| IBIS file stm32u535_545_wlcsp56_smps.ibs
[IBIS ver] 4.2
[File name] stm32u535_545_wlcsp56_smps.ibs
[File Rev] rev1.0
[Date]  11-09-2023
[Source] Data Created at STMicroelectronics
[Notes]  File originated from ELDO simulations.
[Disclaimer]  This information is for modeling purpose only and is
   not guaranteed. The information is subject to change without
   notice.
[Copyright] Copyright 2023 STMicroelectronics Inc.
|   Component stm32u535_545_wlcsp56_smps
[Component] stm32u535_545_wlcsp56_smps
[Manufacturer] STMicroelectronics
[Package]
| variable   typ   min   max
R_pkg  0  NA  NA
L_pkg  0  NA  NA
C_pkg  0  NA  NA
[Pin]   signal_name   model_name
A1  VDDUSB  power
A3  PA15  io8_100m_ft
A5  PA14  io8_100m_ft
A7  PB5  io8_166m_hslv_ft
A9  PB8  io8_100m_hslv_i2c_ft
A11  VDD11  nc
A13  VDD  power
B2  VSS  gnd
B4  PB3  io8_100m_i2c_ft
B6  PB4  io8_100m_i2c_ft
B8  PH3-BOOT0  io8_100m_ft
B10  VSS  gnd
B12  PE4  io8_100m_hslv_tamp_ft
B14  VBAT  power
C1  PA11  io8_usb_ft
C3  PA12  io8_usb_ft
C5  PA13  io8_100m_ft
C7  PB6  io8_100m_i2c_ft
C9  PB9  io8_100m_hslv_i2c_ft
C11  PE3  io8_100m_hslv_tamp_ft
C13  PC14-OSC32_IN  io8_100m_tamp_ft
D2  PA9  io8_100m_ft
D4  PA10  io8_100m_ft
D6  PA3  io8_166m_hslv_ft
D8  PB7  io8_166m_hslv_i2c_ft
D10  PE5  io8_100m_hslv_tamp_ft
D12  PC13  io8_100m_ft_v33
D14  PC15-OSC32_OUT   io8_100m_tamp_ft
E1  PB14  io8_100m_i2c_ft
E3  PB12  io8_166m_hslv_ft
E5  PA8  io8_166m_hslv_ft
E7  PA2  io8_100m_hslv_ft
E9  NRST  nc
E11  PH1-OSC_OUT  io8_100m_ft
E13  PH0-OSC_IN  io8_100m_ft
F2  PB15  io8_100m_ft
F4  PB1  io8_100m_hslv_ft
F6  PB0  io8_100m_hslv_ft
F8  PA5  io8_100m_ft
F10  PA0  io8_100m_hslv_tamp_ft
F12  VDDA  power
F14  VSSA  nc
G1  PB13  io8_100m_i2c_ft
G3  VSS  gnd
G5  VSSSMPS  nc
G7  PB2  io8_100m_hslv_tamp_ft
G9  PA6  io8_100m_hslv_ft
G11  PA4  io8_100m_hslv_ft
G13  PA1  io8_100m_hslv_tamp_ft
H2  VDD  power
H4  VDD11  nc
H6  VDDSMPS  nc
H8  VLXSMPS  nc
H10  PA7  io8_100m_hslv_i2c_ft
H12  VDD  power
H14  VSS  gnd
[Package Model]   455-wlcsp-56-100mhz-230421
[Pin Mapping]   pulldown_ref   pullup_ref   | Comment
A1  nc  vddiom
A3  gndio  vddiom
A5  gndio  vddiom
A7  gndio  vddiom
A9  gndio  vddiom
A11  nc  nc
A13  nc  vddiom
B2  gndio  nc
B4  gndio  vddiom
B6  gndio  vddiom
B8  gndio  vddiom
B10  gndio  nc
B12  gndio  vddiom
B14  nc  vsw
C1  gndio  vddiom
C3  gndio  vddiom
C5  gndio  vddiom
C7  gndio  vddiom
C9  gndio  vddiom
C11  gndio  vddiom
C13  gndio  vddiom  | Depending on IO usage
| C13  gndio  vsw  | Depending on IO usage
D2  gndio  vddiom
D4  gndio  vddiom
D6  gndio  vddiom
D8  gndio  vddiom
D10  gndio  vddiom
D12  gndio  vddiom  | Depending on IO usage
| D12  gndio  vsw  | Depending on IO usage
D14  gndio  vddiom  | Depending on IO usage
| D14  gndio  vsw  | Depending on IO usage
E1  gndio  vddiom
E3  gndio  vddiom
E5  gndio  vddiom
E7  gndio  vddiom
E9  nc   nc
E11  gndio  vddiom
E13  gndio  vddiom
F2  gndio  vddiom
F4  gndio  vddiom
F6  gndio  vddiom
F8  gndio  vddiom
F10  gndio  vddiom
F12  nc  vddiom
F14  nc  nc
G1  gndio  vddiom
G3  gndio  nc
G5  nc  nc
G7  gndio  vddiom
G9  gndio  vddiom
G11  gndio  vddiom
G13  gndio  vddiom
H2  nc  vddiom
H4  nc  nc
H6  nc  nc
H8  nc  nc
H10  gndio  vddiom
H12  nc  vddiom
H14  gndio  nc
[Model Selector] io8_100m_ft
io8_100m_ft_hs_1v2  "IO8_FT 100MHz high speed @ 1.2V"
io8_100m_ft_fs_1v2  "IO8_FT 100MHz fast speed @ 1.2V"
io8_100m_ft_fs_pd_1v2  "IO8_FT 100MHz fast speed @ 1.2V pulldown"
io8_100m_ft_ms_1v2  "IO8_FT 100MHz med speed @ 1.2V"
io8_100m_ft_ms_pd_1v2  "IO8_FT 100MHz med speed @ 1.2V pulldown"
io8_100m_ft_ls_1v2  "IO8_FT 100MHz low speed @ 1.2V"
io8_100m_ft_ls_pd_1v2  "IO8_FT 100MHz low speed @ 1.2V pulldown"
io8_100m_ft_hs_1v8  "IO8_FT 100MHz high speed @ 1.8V"
io8_100m_ft_hs_pd_1v8  "IO8_FT 100MHz high speed @ 1.8V pulldown"
io8_100m_ft_fs_1v8  "IO8_FT 100MHz fast speed @ 1.8V"
io8_100m_ft_fs_pd_1v8  "IO8_FT 100MHz fast speed @ 1.8V pulldown"
io8_100m_ft_ms_1v8  "IO8_FT 100MHz med speed @ 1.8V"
io8_100m_ft_ms_pd_1v8  "IO8_FT 100MHz med speed @ 1.8V pulldown"
io8_100m_ft_ls_1v8  "IO8_FT 100MHz low speed @ 1.8V"
io8_100m_ft_ls_pd_1v8  "IO8_FT 100MHz low speed @ 1.8V pulldown"
io8_100m_ft_hs_3v3  "IO8_FT 100MHz high speed @ 3.3V"
io8_100m_ft_hs_pd_3v3  "IO8_FT 100MHz high speed @ 3.3V pulldown"
io8_100m_ft_fs_3v3  "IO8_FT 100MHz fast speed @ 3.3V"
io8_100m_ft_fs_pd_3v3  "IO8_FT 100MHz fast speed @ 3.3V pulldown"
io8_100m_ft_ms_3v3  "IO8_FT 100MHz med speed @ 3.3V"
io8_100m_ft_ms_pd_3v3  "IO8_FT 100MHz med speed @ 3.3V pulldown"
io8_100m_ft_ls_3v3  "IO8_FT 100MHz low speed @ 3.3V"
io8_100m_ft_ls_pd_3v3  "IO8_FT 100MHz low speed @ 3.3V pulldown"
[Model Selector] io8_100m_hslv_ft
io8_100m_ft_hs_1v2  "IO8_FT 100MHz high speed @ 1.2V"
io8_100m_ft_hs_pu_1v2  "IO8_FT 100MHz high speed @ 1.2V pullup"
io8_100m_ft_hs_pd_1v2  "IO8_FT 100MHz high speed @ 1.2V pulldown"
io8_100m_ft_fs_1v2  "IO8_FT 100MHz fast speed @ 1.2V"
io8_100m_ft_fs_pu_1v2  "IO8_FT 100MHz fast speed @ 1.2V pullup"
io8_100m_ft_fs_pd_1v2  "IO8_FT 100MHz fast speed @ 1.2V pulldown"
io8_100m_ft_ms_1v2  "IO8_FT 100MHz med speed @ 1.2V"
io8_100m_ft_ms_pu_1v2  "IO8_FT 100MHz med speed @ 1.2V pullup"
io8_100m_ft_ms_pd_1v2  "IO8_FT 100MHz med speed @ 1.2V pulldown"
io8_100m_ft_ls_1v2  "IO8_FT 100MHz low speed @ 1.2V"
io8_100m_ft_ls_pu_1v2  "IO8_FT 100MHz low speed @ 1.2V pullup"
io8_100m_ft_ls_pd_1v2  "IO8_FT 100MHz low speed @ 1.2V pulldown"
io8_100m_ft_hs_1v8  "IO8_FT 100MHz high speed @ 1.8V"
io8_100m_ft_hs_pu_1v8  "IO8_FT 100MHz high speed @ 1.8V pullup"
io8_100m_ft_hs_pd_1v8  "IO8_FT 100MHz high speed @ 1.8V pulldown"
io8_100m_ft_fs_1v8  "IO8_FT 100MHz fast speed @ 1.8V"
io8_100m_ft_fs_pu_1v8  "IO8_FT 100MHz fast speed @ 1.8V pullup"
io8_100m_ft_fs_pd_1v8  "IO8_FT 100MHz fast speed @ 1.8V pulldown"
io8_100m_ft_ms_1v8  "IO8_FT 100MHz med speed @ 1.8V"
io8_100m_ft_ms_pu_1v8  "IO8_FT 100MHz med speed @ 1.8V pullup"
io8_100m_ft_ms_pd_1v8  "IO8_FT 100MHz med speed @ 1.8V pulldown"
io8_100m_ft_ls_1v8  "IO8_FT 100MHz low speed @ 1.8V"
io8_100m_ft_ls_pu_1v8  "IO8_FT 100MHz low speed @ 1.8V pullup"
io8_100m_ft_ls_pd_1v8  "IO8_FT 100MHz low speed @ 1.8V pulldown"
io8_100m_ft_hs_3v3  "IO8_FT 100MHz high speed @ 3.3V"
io8_100m_ft_hs_pu_3v3  "IO8_FT 100MHz high speed @ 3.3V pullup"
io8_100m_ft_hs_pd_3v3  "IO8_FT 100MHz high speed @ 3.3V pulldown"
io8_100m_ft_fs_3v3  "IO8_FT 100MHz fast speed @ 3.3V"
io8_100m_ft_fs_pu_3v3  "IO8_FT 100MHz fast speed @ 3.3V pullup"
io8_100m_ft_fs_pd_3v3  "IO8_FT 100MHz fast speed @ 3.3V pulldown"
io8_100m_ft_ms_3v3  "IO8_FT 100MHz med speed @ 3.3V"
io8_100m_ft_ms_pu_3v3  "IO8_FT 100MHz med speed @ 3.3V pullup"
io8_100m_ft_ms_pd_3v3  "IO8_FT 100MHz med speed @ 3.3V pulldown"
io8_100m_ft_ls_3v3  "IO8_FT 100MHz low speed @ 3.3V"
io8_100m_ft_ls_pu_3v3  "IO8_FT 100MHz low speed @ 3.3V pullup"
io8_100m_ft_ls_pd_3v3  "IO8_FT 100MHz low speed @ 3.3V pulldown"
io8_100m_hslv_ft_hs_1v2  "IO8_FT 100MHz HSLV high speed @ 1.2V"
io8_100m_hslv_ft_hs_pu_1v2  "IO8_FT 100MHz HSLV high speed @ 1.2V pullup"
io8_100m_hslv_ft_hs_pd_1v2  "IO8_FT 100MHz HSLV high speed @ 1.2V pulldown"
io8_100m_hslv_ft_fs_1v2  "IO8_FT 100MHz HSLV fast speed @ 1.2V"
io8_100m_hslv_ft_fs_pu_1v2  "IO8_FT 100MHz HSLV fast speed @ 1.2V pullup"
io8_100m_hslv_ft_fs_pd_1v2  "IO8_FT 100MHz HSLV fast speed @ 1.2V pulldown"
io8_100m_hslv_ft_ms_1v2  "IO8_FT 100MHz HSLV med speed @ 1.2V"
io8_100m_hslv_ft_ms_pu_1v2  "IO8_FT 100MHz HSLV med speed @ 1.2V pullup"
io8_100m_hslv_ft_ms_pd_1v2  "IO8_FT 100MHz HSLV med speed @ 1.2V pulldown"
io8_100m_hslv_ft_ls_1v2  "IO8_FT 100MHz HSLV low speed @ 1.2V"
io8_100m_hslv_ft_ls_pu_1v2  "IO8_FT 100MHz HSLV low speed @ 1.2V pullup"
io8_100m_hslv_ft_ls_pd_1v2  "IO8_FT 100MHz HSLV low speed @ 1.2V pulldown"
io8_100m_hslv_ft_hs_1v8  "IO8_FT 100MHz HSLV high speed @ 1.8V"
io8_100m_hslv_ft_hs_pu_1v8  "IO8_FT 100MHz HSLV high speed @ 1.8V pullup"
io8_100m_hslv_ft_hs_pd_1v8  "IO8_FT 100MHz HSLV high speed @ 1.8V pulldown"
io8_100m_hslv_ft_fs_1v8  "IO8_FT 100MHz HSLV fast speed @ 1.8V"
io8_100m_hslv_ft_fs_pu_1v8  "IO8_FT 100MHz HSLV fast speed @ 1.8V pullup"
io8_100m_hslv_ft_fs_pd_1v8  "IO8_FT 100MHz HSLV fast speed @ 1.8V pulldown"
io8_100m_hslv_ft_ms_1v8  "IO8_FT 100MHz HSLV med speed @ 1.8V"
io8_100m_hslv_ft_ms_pu_1v8  "IO8_FT 100MHz HSLV med speed @ 1.8V pullup"
io8_100m_hslv_ft_ms_pd_1v8  "IO8_FT 100MHz HSLV med speed @ 1.8V pulldown"
io8_100m_hslv_ft_ls_1v8  "IO8_FT 100MHz HSLV low speed @ 1.8V"
io8_100m_hslv_ft_ls_pu_1v8  "IO8_FT 100MHz HSLV low speed @ 1.8V pullup"
io8_100m_hslv_ft_ls_pd_1v8  "IO8_FT 100MHz HSLV low speed @ 1.8V pulldown"
io8_100m_hslv_ft_hs_2v5  "IO8_FT 100MHz HSLV high speed @ 2.5V"
io8_100m_hslv_ft_hs_pu_2v5  "IO8_FT 100MHz HSLV high speed @ 2.5V pullup"
io8_100m_hslv_ft_hs_pd_2v5  "IO8_FT 100MHz HSLV high speed @ 2.5V pulldown"
io8_100m_hslv_ft_fs_2v5  "IO8_FT 100MHz HSLV fast speed @ 2.5V"
io8_100m_hslv_ft_fs_pu_2v5  "IO8_FT 100MHz HSLV fast speed @ 2.5V pullup"
io8_100m_hslv_ft_fs_pd_2v5  "IO8_FT 100MHz HSLV fast speed @ 2.5V pulldown"
io8_100m_hslv_ft_ms_2v5  "IO8_FT 100MHz HSLV med speed @ 2.5V"
io8_100m_hslv_ft_ms_pu_2v5  "IO8_FT 100MHz HSLV med speed @ 2.5V pullup"
io8_100m_hslv_ft_ms_pd_2v5  "IO8_FT 100MHz HSLV med speed @ 2.5V pulldown"
io8_100m_hslv_ft_ls_2v5  "IO8_FT 100MHz HSLV low speed @ 2.5V"
io8_100m_hslv_ft_ls_pu_2v5  "IO8_FT 100MHz HSLV low speed @ 2.5V pullup"
io8_100m_hslv_ft_ls_pd_2v5  "IO8_FT 100MHz HSLV low speed @ 2.5V pulldown"
[Model Selector] io8_100m_hslv_i2c_ft
io8_100m_ft_hs_1v2  "IO8_FT 100MHz high speed @ 1.2V"
io8_100m_ft_hs_pu_1v2  "IO8_FT 100MHz high speed @ 1.2V pullup"
io8_100m_ft_hs_pd_1v2  "IO8_FT 100MHz high speed @ 1.2V pulldown"
io8_100m_ft_fs_1v2  "IO8_FT 100MHz fast speed @ 1.2V"
io8_100m_ft_fs_pu_1v2  "IO8_FT 100MHz fast speed @ 1.2V pullup"
io8_100m_ft_fs_pd_1v2  "IO8_FT 100MHz fast speed @ 1.2V pulldown"
io8_100m_ft_ms_1v2  "IO8_FT 100MHz med speed @ 1.2V"
io8_100m_ft_ms_pu_1v2  "IO8_FT 100MHz med speed @ 1.2V pullup"
io8_100m_ft_ms_pd_1v2  "IO8_FT 100MHz med speed @ 1.2V pulldown"
io8_100m_ft_ls_1v2  "IO8_FT 100MHz low speed @ 1.2V"
io8_100m_ft_ls_pu_1v2  "IO8_FT 100MHz low speed @ 1.2V pullup"
io8_100m_ft_ls_pd_1v2  "IO8_FT 100MHz low speed @ 1.2V pulldown"
io8_100m_ft_hs_1v8  "IO8_FT 100MHz high speed @ 1.8V"
io8_100m_ft_hs_pu_1v8  "IO8_FT 100MHz high speed @ 1.8V pullup"
io8_100m_ft_hs_pd_1v8  "IO8_FT 100MHz high speed @ 1.8V pulldown"
io8_100m_ft_fs_1v8  "IO8_FT 100MHz fast speed @ 1.8V"
io8_100m_ft_fs_pu_1v8  "IO8_FT 100MHz fast speed @ 1.8V pullup"
io8_100m_ft_fs_pd_1v8  "IO8_FT 100MHz fast speed @ 1.8V pulldown"
io8_100m_ft_ms_1v8  "IO8_FT 100MHz med speed @ 1.8V"
io8_100m_ft_ms_pu_1v8  "IO8_FT 100MHz med speed @ 1.8V pullup"
io8_100m_ft_ms_pd_1v8  "IO8_FT 100MHz med speed @ 1.8V pulldown"
io8_100m_ft_ls_1v8  "IO8_FT 100MHz low speed @ 1.8V"
io8_100m_ft_ls_pu_1v8  "IO8_FT 100MHz low speed @ 1.8V pullup"
io8_100m_ft_ls_pd_1v8  "IO8_FT 100MHz low speed @ 1.8V pulldown"
io8_100m_ft_hs_3v3  "IO8_FT 100MHz high speed @ 3.3V"
io8_100m_ft_hs_pu_3v3  "IO8_FT 100MHz high speed @ 3.3V pullup"
io8_100m_ft_hs_pd_3v3  "IO8_FT 100MHz high speed @ 3.3V pulldown"
io8_100m_ft_fs_3v3  "IO8_FT 100MHz fast speed @ 3.3V"
io8_100m_ft_fs_pu_3v3  "IO8_FT 100MHz fast speed @ 3.3V pullup"
io8_100m_ft_fs_pd_3v3  "IO8_FT 100MHz fast speed @ 3.3V pulldown"
io8_100m_ft_ms_3v3  "IO8_FT 100MHz med speed @ 3.3V"
io8_100m_ft_ms_pu_3v3  "IO8_FT 100MHz med speed @ 3.3V pullup"
io8_100m_ft_ms_pd_3v3  "IO8_FT 100MHz med speed @ 3.3V pulldown"
io8_100m_ft_ls_3v3  "IO8_FT 100MHz low speed @ 3.3V"
io8_100m_ft_ls_pu_3v3  "IO8_FT 100MHz low speed @ 3.3V pullup"
io8_100m_ft_ls_pd_3v3  "IO8_FT 100MHz low speed @ 3.3V pulldown"
io8_100m_hslv_ft_hs_1v2  "IO8_FT 100MHz HSLV high speed @ 1.2V"
io8_100m_hslv_ft_hs_pu_1v2  "IO8_FT 100MHz HSLV high speed @ 1.2V pullup"
io8_100m_hslv_ft_hs_pd_1v2  "IO8_FT 100MHz HSLV high speed @ 1.2V pulldown"
io8_100m_hslv_ft_fs_1v2  "IO8_FT 100MHz HSLV fast speed @ 1.2V"
io8_100m_hslv_ft_fs_pu_1v2  "IO8_FT 100MHz HSLV fast speed @ 1.2V pullup"
io8_100m_hslv_ft_fs_pd_1v2  "IO8_FT 100MHz HSLV fast speed @ 1.2V pulldown"
io8_100m_hslv_ft_ms_1v2  "IO8_FT 100MHz HSLV med speed @ 1.2V"
io8_100m_hslv_ft_ms_pu_1v2  "IO8_FT 100MHz HSLV med speed @ 1.2V pullup"
io8_100m_hslv_ft_ms_pd_1v2  "IO8_FT 100MHz HSLV med speed @ 1.2V pulldown"
io8_100m_hslv_ft_ls_1v2  "IO8_FT 100MHz HSLV low speed @ 1.2V"
io8_100m_hslv_ft_ls_pu_1v2  "IO8_FT 100MHz HSLV low speed @ 1.2V pullup"
io8_100m_hslv_ft_ls_pd_1v2  "IO8_FT 100MHz HSLV low speed @ 1.2V pulldown"
io8_100m_hslv_ft_hs_1v8  "IO8_FT 100MHz HSLV high speed @ 1.8V"
io8_100m_hslv_ft_hs_pu_1v8  "IO8_FT 100MHz HSLV high speed @ 1.8V pullup"
io8_100m_hslv_ft_hs_pd_1v8  "IO8_FT 100MHz HSLV high speed @ 1.8V pulldown"
io8_100m_hslv_ft_fs_1v8  "IO8_FT 100MHz HSLV fast speed @ 1.8V"
io8_100m_hslv_ft_fs_pu_1v8  "IO8_FT 100MHz HSLV fast speed @ 1.8V pullup"
io8_100m_hslv_ft_fs_pd_1v8  "IO8_FT 100MHz HSLV fast speed @ 1.8V pulldown"
io8_100m_hslv_ft_ms_1v8  "IO8_FT 100MHz HSLV med speed @ 1.8V"
io8_100m_hslv_ft_ms_pu_1v8  "IO8_FT 100MHz HSLV med speed @ 1.8V pullup"
io8_100m_hslv_ft_ms_pd_1v8  "IO8_FT 100MHz HSLV med speed @ 1.8V pulldown"
io8_100m_hslv_ft_ls_1v8  "IO8_FT 100MHz HSLV low speed @ 1.8V"
io8_100m_hslv_ft_ls_pu_1v8  "IO8_FT 100MHz HSLV low speed @ 1.8V pullup"
io8_100m_hslv_ft_ls_pd_1v8  "IO8_FT 100MHz HSLV low speed @ 1.8V pulldown"
io8_100m_hslv_ft_hs_2v5  "IO8_FT 100MHz HSLV high speed @ 2.5V"
io8_100m_hslv_ft_hs_pu_2v5  "IO8_FT 100MHz HSLV high speed @ 2.5V pullup"
io8_100m_hslv_ft_hs_pd_2v5  "IO8_FT 100MHz HSLV high speed @ 2.5V pulldown"
io8_100m_hslv_ft_fs_2v5  "IO8_FT 100MHz HSLV fast speed @ 2.5V"
io8_100m_hslv_ft_fs_pu_2v5  "IO8_FT 100MHz HSLV fast speed @ 2.5V pullup"
io8_100m_hslv_ft_fs_pd_2v5  "IO8_FT 100MHz HSLV fast speed @ 2.5V pulldown"
io8_100m_hslv_ft_ms_2v5  "IO8_FT 100MHz HSLV med speed @ 2.5V"
io8_100m_hslv_ft_ms_pu_2v5  "IO8_FT 100MHz HSLV med speed @ 2.5V pullup"
io8_100m_hslv_ft_ms_pd_2v5  "IO8_FT 100MHz HSLV med speed @ 2.5V pulldown"
io8_100m_hslv_ft_ls_2v5  "IO8_FT 100MHz HSLV low speed @ 2.5V"
io8_100m_hslv_ft_ls_pu_2v5  "IO8_FT 100MHz HSLV low speed @ 2.5V pullup"
io8_100m_hslv_ft_ls_pd_2v5  "IO8_FT 100MHz HSLV low speed @ 2.5V pulldown"
[Model Selector] io8_100m_hslv_tamp_ft
io8_100m_ft_hs_1v2  "IO8_FT 100MHz high speed @ 1.2V"
io8_100m_ft_hs_pu_1v2  "IO8_FT 100MHz high speed @ 1.2V pullup"
io8_100m_ft_hs_pd_1v2  "IO8_FT 100MHz high speed @ 1.2V pulldown"
io8_100m_ft_fs_1v2  "IO8_FT 100MHz fast speed @ 1.2V"
io8_100m_ft_fs_pu_1v2  "IO8_FT 100MHz fast speed @ 1.2V pullup"
io8_100m_ft_fs_pd_1v2  "IO8_FT 100MHz fast speed @ 1.2V pulldown"
io8_100m_ft_ms_1v2  "IO8_FT 100MHz med speed @ 1.2V"
io8_100m_ft_ms_pu_1v2  "IO8_FT 100MHz med speed @ 1.2V pullup"
io8_100m_ft_ms_pd_1v2  "IO8_FT 100MHz med speed @ 1.2V pulldown"
io8_100m_ft_ls_1v2  "IO8_FT 100MHz low speed @ 1.2V"
io8_100m_ft_ls_pu_1v2  "IO8_FT 100MHz low speed @ 1.2V pullup"
io8_100m_ft_ls_pd_1v2  "IO8_FT 100MHz low speed @ 1.2V pulldown"
io8_100m_ft_hs_1v8  "IO8_FT 100MHz high speed @ 1.8V"
io8_100m_ft_hs_pu_1v8  "IO8_FT 100MHz high speed @ 1.8V pullup"
io8_100m_ft_hs_pd_1v8  "IO8_FT 100MHz high speed @ 1.8V pulldown"
io8_100m_ft_fs_1v8  "IO8_FT 100MHz fast speed @ 1.8V"
io8_100m_ft_fs_pu_1v8  "IO8_FT 100MHz fast speed @ 1.8V pullup"
io8_100m_ft_fs_pd_1v8  "IO8_FT 100MHz fast speed @ 1.8V pulldown"
io8_100m_ft_ms_1v8  "IO8_FT 100MHz med speed @ 1.8V"
io8_100m_ft_ms_pu_1v8  "IO8_FT 100MHz med speed @ 1.8V pullup"
io8_100m_ft_ms_pd_1v8  "IO8_FT 100MHz med speed @ 1.8V pulldown"
io8_100m_ft_ls_1v8  "IO8_FT 100MHz low speed @ 1.8V"
io8_100m_ft_ls_pu_1v8  "IO8_FT 100MHz low speed @ 1.8V pullup"
io8_100m_ft_ls_pd_1v8  "IO8_FT 100MHz low speed @ 1.8V pulldown"
io8_100m_ft_hs_3v3  "IO8_FT 100MHz high speed @ 3.3V"
io8_100m_ft_hs_pu_3v3  "IO8_FT 100MHz high speed @ 3.3V pullup"
io8_100m_ft_hs_pd_3v3  "IO8_FT 100MHz high speed @ 3.3V pulldown"
io8_100m_ft_fs_3v3  "IO8_FT 100MHz fast speed @ 3.3V"
io8_100m_ft_fs_pu_3v3  "IO8_FT 100MHz fast speed @ 3.3V pullup"
io8_100m_ft_fs_pd_3v3  "IO8_FT 100MHz fast speed @ 3.3V pulldown"
io8_100m_ft_ms_3v3  "IO8_FT 100MHz med speed @ 3.3V"
io8_100m_ft_ms_pu_3v3  "IO8_FT 100MHz med speed @ 3.3V pullup"
io8_100m_ft_ms_pd_3v3  "IO8_FT 100MHz med speed @ 3.3V pulldown"
io8_100m_ft_ls_3v3  "IO8_FT 100MHz low speed @ 3.3V"
io8_100m_ft_ls_pu_3v3  "IO8_FT 100MHz low speed @ 3.3V pullup"
io8_100m_ft_ls_pd_3v3  "IO8_FT 100MHz low speed @ 3.3V pulldown"
io8_100m_hslv_ft_hs_1v2  "IO8_FT 100MHz HSLV high speed @ 1.2V"
io8_100m_hslv_ft_hs_pu_1v2  "IO8_FT 100MHz HSLV high speed @ 1.2V pullup"
io8_100m_hslv_ft_hs_pd_1v2  "IO8_FT 100MHz HSLV high speed @ 1.2V pulldown"
io8_100m_hslv_ft_fs_1v2  "IO8_FT 100MHz HSLV fast speed @ 1.2V"
io8_100m_hslv_ft_fs_pu_1v2  "IO8_FT 100MHz HSLV fast speed @ 1.2V pullup"
io8_100m_hslv_ft_fs_pd_1v2  "IO8_FT 100MHz HSLV fast speed @ 1.2V pulldown"
io8_100m_hslv_ft_ms_1v2  "IO8_FT 100MHz HSLV med speed @ 1.2V"
io8_100m_hslv_ft_ms_pu_1v2  "IO8_FT 100MHz HSLV med speed @ 1.2V pullup"
io8_100m_hslv_ft_ms_pd_1v2  "IO8_FT 100MHz HSLV med speed @ 1.2V pulldown"
io8_100m_hslv_ft_ls_1v2  "IO8_FT 100MHz HSLV low speed @ 1.2V"
io8_100m_hslv_ft_ls_pu_1v2  "IO8_FT 100MHz HSLV low speed @ 1.2V pullup"
io8_100m_hslv_ft_ls_pd_1v2  "IO8_FT 100MHz HSLV low speed @ 1.2V pulldown"
io8_100m_hslv_ft_hs_1v8  "IO8_FT 100MHz HSLV high speed @ 1.8V"
io8_100m_hslv_ft_hs_pu_1v8  "IO8_FT 100MHz HSLV high speed @ 1.8V pullup"
io8_100m_hslv_ft_hs_pd_1v8  "IO8_FT 100MHz HSLV high speed @ 1.8V pulldown"
io8_100m_hslv_ft_fs_1v8  "IO8_FT 100MHz HSLV fast speed @ 1.8V"
io8_100m_hslv_ft_fs_pu_1v8  "IO8_FT 100MHz HSLV fast speed @ 1.8V pullup"
io8_100m_hslv_ft_fs_pd_1v8  "IO8_FT 100MHz HSLV fast speed @ 1.8V pulldown"
io8_100m_hslv_ft_ms_1v8  "IO8_FT 100MHz HSLV med speed @ 1.8V"
io8_100m_hslv_ft_ms_pu_1v8  "IO8_FT 100MHz HSLV med speed @ 1.8V pullup"
io8_100m_hslv_ft_ms_pd_1v8  "IO8_FT 100MHz HSLV med speed @ 1.8V pulldown"
io8_100m_hslv_ft_ls_1v8  "IO8_FT 100MHz HSLV low speed @ 1.8V"
io8_100m_hslv_ft_ls_pu_1v8  "IO8_FT 100MHz HSLV low speed @ 1.8V pullup"
io8_100m_hslv_ft_ls_pd_1v8  "IO8_FT 100MHz HSLV low speed @ 1.8V pulldown"
io8_100m_hslv_ft_hs_2v5  "IO8_FT 100MHz HSLV high speed @ 2.5V"
io8_100m_hslv_ft_hs_pu_2v5  "IO8_FT 100MHz HSLV high speed @ 2.5V pullup"
io8_100m_hslv_ft_hs_pd_2v5  "IO8_FT 100MHz HSLV high speed @ 2.5V pulldown"
io8_100m_hslv_ft_fs_2v5  "IO8_FT 100MHz HSLV fast speed @ 2.5V"
io8_100m_hslv_ft_fs_pu_2v5  "IO8_FT 100MHz HSLV fast speed @ 2.5V pullup"
io8_100m_hslv_ft_fs_pd_2v5  "IO8_FT 100MHz HSLV fast speed @ 2.5V pulldown"
io8_100m_hslv_ft_ms_2v5  "IO8_FT 100MHz HSLV med speed @ 2.5V"
io8_100m_hslv_ft_ms_pu_2v5  "IO8_FT 100MHz HSLV med speed @ 2.5V pullup"
io8_100m_hslv_ft_ms_pd_2v5  "IO8_FT 100MHz HSLV med speed @ 2.5V pulldown"
io8_100m_hslv_ft_ls_2v5  "IO8_FT 100MHz HSLV low speed @ 2.5V"
io8_100m_hslv_ft_ls_pu_2v5  "IO8_FT 100MHz HSLV low speed @ 2.5V pullup"
io8_100m_hslv_ft_ls_pd_2v5  "IO8_FT 100MHz HSLV low speed @ 2.5V pulldown"
io8_ft_v33_hs_1v2  "IO8_FT_V33 high speed @ 1.2V"
io8_ft_v33_hs_pu_1v2  "IO8_FT_V33 high speed @ 1.2V pullup"
io8_ft_v33_hs_pd_1v2  "IO8_FT_V33 high speed @ 1.2V pulldown"
io8_ft_v33_fs_1v2  "IO8_FT_V33 fast speed @ 1.2V"
io8_ft_v33_fs_pu_1v2  "IO8_FT_V33 fast speed @ 1.2V pullup"
io8_ft_v33_fs_pd_1v2  "IO8_FT_V33 fast speed @ 1.2V pulldown"
io8_ft_v33_ms_1v2  "IO8_FT_V33 med speed @ 1.2V"
io8_ft_v33_ms_pu_1v2  "IO8_FT_V33 med speed @ 1.2V pullup"
io8_ft_v33_ms_pd_1v2  "IO8_FT_V33 med speed @ 1.2V pulldown"
io8_ft_v33_ls_1v2  "IO8_FT_V33 low speed @ 1.2V"
io8_ft_v33_ls_pu_1v2  "IO8_FT_V33 low speed @ 1.2V pullup"
io8_ft_v33_ls_pd_1v2  "IO8_FT_V33 low speed @ 1.2V pulldown"
io8_ft_v33_hs_1v8  "IO8_FT_V33 high speed @ 1.8V"
io8_ft_v33_hs_pu_1v8  "IO8_FT_V33 high speed @ 1.8V pullup"
io8_ft_v33_hs_pd_1v8  "IO8_FT_V33 high speed @ 1.8V pulldown"
io8_ft_v33_fs_1v8  "IO8_FT_V33 fast speed @ 1.8V"
io8_ft_v33_fs_pu_1v8  "IO8_FT_V33 fast speed @ 1.8V pullup"
io8_ft_v33_fs_pd_1v8  "IO8_FT_V33 fast speed @ 1.8V pulldown"
io8_ft_v33_ms_1v8  "IO8_FT_V33 med speed @ 1.8V"
io8_ft_v33_ms_pu_1v8  "IO8_FT_V33 med speed @ 1.8V pullup"
io8_ft_v33_ms_pd_1v8  "IO8_FT_V33 med speed @ 1.8V pulldown"
io8_ft_v33_ls_1v8  "IO8_FT_V33 low speed @ 1.8V"
io8_ft_v33_ls_pu_1v8  "IO8_FT_V33 low speed @ 1.8V pullup"
io8_ft_v33_ls_pd_1v8  "IO8_FT_V33 low speed @ 1.8V pulldown"
io8_ft_v33_hs_3v3  "IO8_FT_V33 high speed @ 3.3V"
io8_ft_v33_hs_pu_3v3  "IO8_FT_V33 high speed @ 3.3V pullup"
io8_ft_v33_hs_pd_3v3  "IO8_FT_V33 high speed @ 3.3V pulldown"
io8_ft_v33_fs_3v3  "IO8_FT_V33 fast speed @ 3.3V"
io8_ft_v33_fs_pu_3v3  "IO8_FT_V33 fast speed @ 3.3V pullup"
io8_ft_v33_fs_pd_3v3  "IO8_FT_V33 fast speed @ 3.3V pulldown"
io8_ft_v33_ms_3v3  "IO8_FT_V33 med speed @ 3.3V"
io8_ft_v33_ms_pu_3v3  "IO8_FT_V33 med speed @ 3.3V pullup"
io8_ft_v33_ms_pd_3v3  "IO8_FT_V33 med speed @ 3.3V pulldown"
io8_ft_v33_ls_3v3  "IO8_FT_V33 low speed @ 3.3V"
io8_ft_v33_ls_pu_3v3  "IO8_FT_V33 low speed @ 3.3V pullup"
io8_ft_v33_ls_pd_3v3  "IO8_FT_V33 low speed @ 3.3V pulldown"
[Model Selector] io8_100m_i2c_ft
io8_100m_ft_hs_1v2  "IO8_FT 100MHz high speed @ 1.2V"
io8_100m_ft_hs_pu_1v2  "IO8_FT 100MHz high speed @ 1.2V pullup"
io8_100m_ft_hs_pd_1v2  "IO8_FT 100MHz high speed @ 1.2V pulldown"
io8_100m_ft_fs_1v2  "IO8_FT 100MHz fast speed @ 1.2V"
io8_100m_ft_fs_pu_1v2  "IO8_FT 100MHz fast speed @ 1.2V pullup"
io8_100m_ft_fs_pd_1v2  "IO8_FT 100MHz fast speed @ 1.2V pulldown"
io8_100m_ft_ms_1v2  "IO8_FT 100MHz med speed @ 1.2V"
io8_100m_ft_ms_pu_1v2  "IO8_FT 100MHz med speed @ 1.2V pullup"
io8_100m_ft_ms_pd_1v2  "IO8_FT 100MHz med speed @ 1.2V pulldown"
io8_100m_ft_ls_1v2  "IO8_FT 100MHz low speed @ 1.2V"
io8_100m_ft_ls_pu_1v2  "IO8_FT 100MHz low speed @ 1.2V pullup"
io8_100m_ft_ls_pd_1v2  "IO8_FT 100MHz low speed @ 1.2V pulldown"
io8_100m_ft_hs_1v8  "IO8_FT 100MHz high speed @ 1.8V"
io8_100m_ft_hs_pu_1v8  "IO8_FT 100MHz high speed @ 1.8V pullup"
io8_100m_ft_hs_pd_1v8  "IO8_FT 100MHz high speed @ 1.8V pulldown"
io8_100m_ft_fs_1v8  "IO8_FT 100MHz fast speed @ 1.8V"
io8_100m_ft_fs_pu_1v8  "IO8_FT 100MHz fast speed @ 1.8V pullup"
io8_100m_ft_fs_pd_1v8  "IO8_FT 100MHz fast speed @ 1.8V pulldown"
io8_100m_ft_ms_1v8  "IO8_FT 100MHz med speed @ 1.8V"
io8_100m_ft_ms_pu_1v8  "IO8_FT 100MHz med speed @ 1.8V pullup"
io8_100m_ft_ms_pd_1v8  "IO8_FT 100MHz med speed @ 1.8V pulldown"
io8_100m_ft_ls_1v8  "IO8_FT 100MHz low speed @ 1.8V"
io8_100m_ft_ls_pu_1v8  "IO8_FT 100MHz low speed @ 1.8V pullup"
io8_100m_ft_ls_pd_1v8  "IO8_FT 100MHz low speed @ 1.8V pulldown"
io8_100m_ft_hs_3v3  "IO8_FT 100MHz high speed @ 3.3V"
io8_100m_ft_hs_pu_3v3  "IO8_FT 100MHz high speed @ 3.3V pullup"
io8_100m_ft_hs_pd_3v3  "IO8_FT 100MHz high speed @ 3.3V pulldown"
io8_100m_ft_fs_3v3  "IO8_FT 100MHz fast speed @ 3.3V"
io8_100m_ft_fs_pu_3v3  "IO8_FT 100MHz fast speed @ 3.3V pullup"
io8_100m_ft_fs_pd_3v3  "IO8_FT 100MHz fast speed @ 3.3V pulldown"
io8_100m_ft_ms_3v3  "IO8_FT 100MHz med speed @ 3.3V"
io8_100m_ft_ms_pu_3v3  "IO8_FT 100MHz med speed @ 3.3V pullup"
io8_100m_ft_ms_pd_3v3  "IO8_FT 100MHz med speed @ 3.3V pulldown"
io8_100m_ft_ls_3v3  "IO8_FT 100MHz low speed @ 3.3V"
io8_100m_ft_ls_pu_3v3  "IO8_FT 100MHz low speed @ 3.3V pullup"
io8_100m_ft_ls_pd_3v3  "IO8_FT 100MHz low speed @ 3.3V pulldown"
io8_100m_i2c_ft_1v2  "IO8_FT 100MHz I2C @ 1.2V"
io8_100m_i2c_ft_pu_1v2  "IO8_FT 100MHz I2C @ 1.2V pullup"
io8_100m_i2c_ft_pd_1v2  "IO8_FT 100MHz I2C @ 1.2V pulldown"
io8_100m_i2c_ft_1v8  "IO8_FT 100MHz I2C @ 1.8V"
io8_100m_i2c_ft_pu_1v8  "IO8_FT 100MHz I2C @ 1.8V pullup"
io8_100m_i2c_ft_pd_1v8  "IO8_FT 100MHz I2C @ 1,8V pulldown"
io8_100m_i2c_ft_3v3  "IO8_FT 100MHz I2C @ 3.3V"
io8_100m_i2c_ft_pu_3v3  "IO8_FT 100MHz I2C HSLV @ 3.3V pullup"
io8_100m_i2c_ft_pd_3v3  "IO8_FT 100MHz I2C @ 3.3V pulldown"
[Model Selector] io8_100m_tamp_ft
io8_100m_ft_hs_1v2  "IO8_FT 100MHz high speed @ 1.2V"
io8_100m_ft_hs_pu_1v2  "IO8_FT 100MHz high speed @ 1.2V pullup"
io8_100m_ft_hs_pd_1v2  "IO8_FT 100MHz high speed @ 1.2V pulldown"
io8_100m_ft_fs_1v2  "IO8_FT 100MHz fast speed @ 1.2V"
io8_100m_ft_fs_pu_1v2  "IO8_FT 100MHz fast speed @ 1.2V pullup"
io8_100m_ft_fs_pd_1v2  "IO8_FT 100MHz fast speed @ 1.2V pulldown"
io8_100m_ft_ms_1v2  "IO8_FT 100MHz med speed @ 1.2V"
io8_100m_ft_ms_pu_1v2  "IO8_FT 100MHz med speed @ 1.2V pullup"
io8_100m_ft_ms_pd_1v2  "IO8_FT 100MHz med speed @ 1.2V pulldown"
io8_100m_ft_ls_1v2  "IO8_FT 100MHz low speed @ 1.2V"
io8_100m_ft_ls_pu_1v2  "IO8_FT 100MHz low speed @ 1.2V pullup"
io8_100m_ft_ls_pd_1v2  "IO8_FT 100MHz low speed @ 1.2V pulldown"
io8_100m_ft_hs_1v8  "IO8_FT 100MHz high speed @ 1.8V"
io8_100m_ft_hs_pu_1v8  "IO8_FT 100MHz high speed @ 1.8V pullup"
io8_100m_ft_hs_pd_1v8  "IO8_FT 100MHz high speed @ 1.8V pulldown"
io8_100m_ft_fs_1v8  "IO8_FT 100MHz fast speed @ 1.8V"
io8_100m_ft_fs_pu_1v8  "IO8_FT 100MHz fast speed @ 1.8V pullup"
io8_100m_ft_fs_pd_1v8  "IO8_FT 100MHz fast speed @ 1.8V pulldown"
io8_100m_ft_ms_1v8  "IO8_FT 100MHz med speed @ 1.8V"
io8_100m_ft_ms_pu_1v8  "IO8_FT 100MHz med speed @ 1.8V pullup"
io8_100m_ft_ms_pd_1v8  "IO8_FT 100MHz med speed @ 1.8V pulldown"
io8_100m_ft_ls_1v8  "IO8_FT 100MHz low speed @ 1.8V"
io8_100m_ft_ls_pu_1v8  "IO8_FT 100MHz low speed @ 1.8V pullup"
io8_100m_ft_ls_pd_1v8  "IO8_FT 100MHz low speed @ 1.8V pulldown"
io8_100m_ft_hs_3v3  "IO8_FT 100MHz high speed @ 3.3V"
io8_100m_ft_hs_pu_3v3  "IO8_FT 100MHz high speed @ 3.3V pullup"
io8_100m_ft_hs_pd_3v3  "IO8_FT 100MHz high speed @ 3.3V pulldown"
io8_100m_ft_fs_3v3  "IO8_FT 100MHz fast speed @ 3.3V"
io8_100m_ft_fs_pu_3v3  "IO8_FT 100MHz fast speed @ 3.3V pullup"
io8_100m_ft_fs_pd_3v3  "IO8_FT 100MHz fast speed @ 3.3V pulldown"
io8_100m_ft_ms_3v3  "IO8_FT 100MHz med speed @ 3.3V"
io8_100m_ft_ms_pu_3v3  "IO8_FT 100MHz med speed @ 3.3V pullup"
io8_100m_ft_ms_pd_3v3  "IO8_FT 100MHz med speed @ 3.3V pulldown"
io8_100m_ft_ls_3v3  "IO8_FT 100MHz low speed @ 3.3V"
io8_100m_ft_ls_pu_3v3  "IO8_FT 100MHz low speed @ 3.3V pullup"
io8_100m_ft_ls_pd_3v3  "IO8_FT 100MHz low speed @ 3.3V pulldown"
io8_ft_v33_hs_1v2  "IO8_FT_V33 high speed @ 1.2V"
io8_ft_v33_hs_pu_1v2  "IO8_FT_V33 high speed @ 1.2V pullup"
io8_ft_v33_hs_pd_1v2  "IO8_FT_V33 high speed @ 1.2V pulldown"
io8_ft_v33_fs_1v2  "IO8_FT_V33 fast speed @ 1.2V"
io8_ft_v33_fs_pu_1v2  "IO8_FT_V33 fast speed @ 1.2V pullup"
io8_ft_v33_fs_pd_1v2  "IO8_FT_V33 fast speed @ 1.2V pulldown"
io8_ft_v33_ms_1v2  "IO8_FT_V33 med speed @ 1.2V"
io8_ft_v33_ms_pu_1v2  "IO8_FT_V33 med speed @ 1.2V pullup"
io8_ft_v33_ms_pd_1v2  "IO8_FT_V33 med speed @ 1.2V pulldown"
io8_ft_v33_ls_1v2  "IO8_FT_V33 low speed @ 1.2V"
io8_ft_v33_ls_pu_1v2  "IO8_FT_V33 low speed @ 1.2V pullup"
io8_ft_v33_ls_pd_1v2  "IO8_FT_V33 low speed @ 1.2V pulldown"
io8_ft_v33_hs_1v8  "IO8_FT_V33 high speed @ 1.8V"
io8_ft_v33_hs_pu_1v8  "IO8_FT_V33 high speed @ 1.8V pullup"
io8_ft_v33_hs_pd_1v8  "IO8_FT_V33 high speed @ 1.8V pulldown"
io8_ft_v33_fs_1v8  "IO8_FT_V33 fast speed @ 1.8V"
io8_ft_v33_fs_pu_1v8  "IO8_FT_V33 fast speed @ 1.8V pullup"
io8_ft_v33_fs_pd_1v8  "IO8_FT_V33 fast speed @ 1.8V pulldown"
io8_ft_v33_ms_1v8  "IO8_FT_V33 med speed @ 1.8V"
io8_ft_v33_ms_pu_1v8  "IO8_FT_V33 med speed @ 1.8V pullup"
io8_ft_v33_ms_pd_1v8  "IO8_FT_V33 med speed @ 1.8V pulldown"
io8_ft_v33_ls_1v8  "IO8_FT_V33 low speed @ 1.8V"
io8_ft_v33_ls_pu_1v8  "IO8_FT_V33 low speed @ 1.8V pullup"
io8_ft_v33_ls_pd_1v8  "IO8_FT_V33 low speed @ 1.8V pulldown"
io8_ft_v33_hs_3v3  "IO8_FT_V33 high speed @ 3.3V"
io8_ft_v33_hs_pu_3v3  "IO8_FT_V33 high speed @ 3.3V pullup"
io8_ft_v33_hs_pd_3v3  "IO8_FT_V33 high speed @ 3.3V pulldown"
io8_ft_v33_fs_3v3  "IO8_FT_V33 fast speed @ 3.3V"
io8_ft_v33_fs_pu_3v3  "IO8_FT_V33 fast speed @ 3.3V pullup"
io8_ft_v33_fs_pd_3v3  "IO8_FT_V33 fast speed @ 3.3V pulldown"
io8_ft_v33_ms_3v3  "IO8_FT_V33 med speed @ 3.3V"
io8_ft_v33_ms_pu_3v3  "IO8_FT_V33 med speed @ 3.3V pullup"
io8_ft_v33_ms_pd_3v3  "IO8_FT_V33 med speed @ 3.3V pulldown"
io8_ft_v33_ls_3v3  "IO8_FT_V33 low speed @ 3.3V"
io8_ft_v33_ls_pu_3v3  "IO8_FT_V33 low speed @ 3.3V pullup"
io8_ft_v33_ls_pd_3v3  "IO8_FT_V33 low speed @ 3.3V pulldown"
[Model Selector] io8_usb_ft
io8_100m_ft_hs_1v2  "IO8_FT 100MHz high speed @ 1.2V"
io8_100m_ft_hs_pu_1v2  "IO8_FT 100MHz high speed @ 1.2V pullup"
io8_100m_ft_hs_pd_1v2  "IO8_FT 100MHz high speed @ 1.2V pulldown"
io8_100m_ft_fs_1v2  "IO8_FT 100MHz fast speed @ 1.2V"
io8_100m_ft_fs_pu_1v2  "IO8_FT 100MHz fast speed @ 1.2V pullup"
io8_100m_ft_fs_pd_1v2  "IO8_FT 100MHz fast speed @ 1.2V pulldown"
io8_100m_ft_ms_1v2  "IO8_FT 100MHz med speed @ 1.2V"
io8_100m_ft_ms_pu_1v2  "IO8_FT 100MHz med speed @ 1.2V pullup"
io8_100m_ft_ms_pd_1v2  "IO8_FT 100MHz med speed @ 1.2V pulldown"
io8_100m_ft_ls_1v2  "IO8_FT 100MHz low speed @ 1.2V"
io8_100m_ft_ls_pu_1v2  "IO8_FT 100MHz low speed @ 1.2V pullup"
io8_100m_ft_ls_pd_1v2  "IO8_FT 100MHz low speed @ 1.2V pulldown"
io8_100m_ft_hs_1v8  "IO8_FT 100MHz high speed @ 1.8V"
io8_100m_ft_hs_pu_1v8  "IO8_FT 100MHz high speed @ 1.8V pullup"
io8_100m_ft_hs_pd_1v8  "IO8_FT 100MHz high speed @ 1.8V pulldown"
io8_100m_ft_fs_1v8  "IO8_FT 100MHz fast speed @ 1.8V"
io8_100m_ft_fs_pu_1v8  "IO8_FT 100MHz fast speed @ 1.8V pullup"
io8_100m_ft_fs_pd_1v8  "IO8_FT 100MHz fast speed @ 1.8V pulldown"
io8_100m_ft_ms_1v8  "IO8_FT 100MHz med speed @ 1.8V"
io8_100m_ft_ms_pu_1v8  "IO8_FT 100MHz med speed @ 1.8V pullup"
io8_100m_ft_ms_pd_1v8  "IO8_FT 100MHz med speed @ 1.8V pulldown"
io8_100m_ft_ls_1v8  "IO8_FT 100MHz low speed @ 1.8V"
io8_100m_ft_ls_pu_1v8  "IO8_FT 100MHz low speed @ 1.8V pullup"
io8_100m_ft_ls_pd_1v8  "IO8_FT 100MHz low speed @ 1.8V pulldown"
io8_100m_ft_hs_3v3  "IO8_FT 100MHz high speed @ 3.3V"
io8_100m_ft_hs_pu_3v3  "IO8_FT 100MHz high speed @ 3.3V pullup"
io8_100m_ft_hs_pd_3v3  "IO8_FT 100MHz high speed @ 3.3V pulldown"
io8_100m_ft_fs_3v3  "IO8_FT 100MHz fast speed @ 3.3V"
io8_100m_ft_fs_pu_3v3  "IO8_FT 100MHz fast speed @ 3.3V pullup"
io8_100m_ft_fs_pd_3v3  "IO8_FT 100MHz fast speed @ 3.3V pulldown"
io8_100m_ft_ms_3v3  "IO8_FT 100MHz med speed @ 3.3V"
io8_100m_ft_ms_pu_3v3  "IO8_FT 100MHz med speed @ 3.3V pullup"
io8_100m_ft_ms_pd_3v3  "IO8_FT 100MHz med speed @ 3.3V pulldown"
io8_100m_ft_ls_3v3  "IO8_FT 100MHz low speed @ 3.3V"
io8_100m_ft_ls_pu_3v3  "IO8_FT 100MHz low speed @ 3.3V pullup"
io8_100m_ft_ls_pd_3v3  "IO8_FT 100MHz low speed @ 3.3V pulldown"
io8_usb_fs_3v3  "IOUSB fast speed @ 3.3V"
io8_usb_fs_pu1_3v3  "IO8USB fast speed @ 3.3V pullup1"
io8_usb_fs_pd1_3v3  "IOUSB fast speed @ 3.3V pulldown1"
io8_usb_ls_3v3  "IOUSB low speed @ 3.3V"
io8_usb_ls_pu1_3v3  "IOUSB low speed @ 3.3V pullup1"
io8_usb_ls_pd1_3v3  "IOUSB low speed @ 3.3V pulldown1"
io8_usb_fs_pu2_3v3  "IOUSB fast speed @ 3.3V pullup2"
io8_usb_fs_pd2_3v3  "IOUSB fast speed @ 3.3V pulldown2"
io8_usb_ls_pu2_3v3  "IOUSB low speed @ 3.3V pullup2"
io8_usb_ls_pd2_3v3  "IOUSB low speed @ 3.3V pulldown2"
[Model Selector] io8_166m_hslv_ft
io8_166m_ft_hs_1v2  "IO8_FT 166MHz high speed @ 1.2V"
io8_166m_ft_hs_pu_1v2  "IO8_FT 166MHz high speed @ 1.2V pullup"
io8_166m_ft_hs_pd_1v2  "IO8_FT 166MHz high speed @ 1.2V pulldown"
io8_166m_ft_fs_1v2  "IO8_FT 166MHz fast speed @ 1.2V"
io8_166m_ft_fs_pu_1v2  "IO8_FT 166MHz fast speed @ 1.2V pullup"
io8_166m_ft_fs_pd_1v2  "IO8_FT 166MHz fast speed @ 1.2V pulldown"
io8_166m_ft_ms_1v2  "IO8_FT 166MHz med speed @ 1.2V"
io8_166m_ft_ms_pu_1v2  "IO8_FT 166MHz med speed @ 1.2V pullup"
io8_166m_ft_ms_pd_1v2  "IO8_FT 166MHz med speed @ 1.2V pulldown"
io8_166m_ft_ls_1v2  "IO8_FT 166MHz low speed @ 1.2V"
io8_166m_ft_ls_pu_1v2  "IO8_FT 166MHz low speed @ 1.2V pullup"
io8_166m_ft_ls_pd_1v2  "IO8_FT 166MHz low speed @ 1.2V pulldown"
io8_166m_ft_hs_1v8  "IO8_FT 166MHz high speed @ 1.8V"
io8_166m_ft_hs_pu_1v8  "IO8_FT 166MHz high speed @ 1.8V pullup"
io8_166m_ft_hs_pd_1v8  "IO8_FT 166MHz high speed @ 1.8V pulldown"
io8_166m_ft_fs_1v8  "IO8_FT 166MHz fast speed @ 1.8V"
io8_166m_ft_fs_pu_1v8  "IO8_FT 166MHz fast speed @ 1.8V pullup"
io8_166m_ft_fs_pd_1v8  "IO8_FT 166MHz fast speed @ 1.8V pulldown"
io8_166m_ft_ms_1v8  "IO8_FT 166MHz med speed @ 1.8V"
io8_166m_ft_ms_pu_1v8  "IO8_FT 166MHz med speed @ 1.8V pullup"
io8_166m_ft_ms_pd_1v8  "IO8_FT 166MHz med speed @ 1.8V pulldown"
io8_166m_ft_ls_1v8  "IO8_FT 166MHz low speed @ 1.8V"
io8_166m_ft_ls_pu_1v8  "IO8_FT 166MHz low speed @ 1.8V pullup"
io8_166m_ft_ls_pd_1v8  "IO8_FT 166MHz low speed @ 1.8V pulldown"
io8_166m_ft_hs_3v3  "IO8_FT 166MHz high speed @ 3.3V"
io8_166m_ft_hs_pu_3v3  "IO8_FT 166MHz high speed @ 3.3V pullup"
io8_166m_ft_hs_pd_3v3  "IO8_FT 166MHz high speed @ 3.3V pulldown"
io8_166m_ft_fs_3v3  "IO8_FT 166MHz fast speed @ 3.3V"
io8_166m_ft_fs_pu_3v3  "IO8_FT 166MHz fast speed @ 3.3V pullup"
io8_166m_ft_fs_pd_3v3  "IO8_FT 166MHz fast speed @ 3.3V pulldown"
io8_166m_ft_ms_3v3  "IO8_FT 166MHz med speed @ 3.3V"
io8_166m_ft_ms_pu_3v3  "IO8_FT 166MHz med speed @ 3.3V pullup"
io8_166m_ft_ms_pd_3v3  "IO8_FT 166MHz med speed @ 3.3V pulldown"
io8_166m_ft_ls_3v3  "IO8_FT 166MHz low speed @ 3.3V"
io8_166m_ft_ls_pu_3v3  "IO8_FT 166MHz low speed @ 3.3V pullup"
io8_166m_ft_ls_pd_3v3  "IO8_FT 166MHz low speed @ 3.3V pulldown"
io8_166m_hslv_ft_hs_1v2  "IO8_FT 166MHz HSLV high speed @ 1.2V"
io8_166m_hslv_ft_hs_pu_1v2  "IO8_FT 166MHz HSLV high speed @ 1.2V pullup"
io8_166m_hslv_ft_hs_pd_1v2  "IO8_FT 166MHz HSLV high speed @ 1.2V pulldown"
io8_166m_hslv_ft_fs_1v2  "IO8_FT 166MHz HSLV fast speed @ 1.2V"
io8_166m_hslv_ft_fs_pu_1v2  "IO8_FT 166MHz HSLV fast speed @ 1.2V pullup"
io8_166m_hslv_ft_fs_pd_1v2  "IO8_FT 166MHz HSLV fast speed @ 1.2V pulldown"
io8_166m_hslv_ft_ms_1v2  "IO8_FT 166MHz HSLV med speed @ 1.2V"
io8_166m_hslv_ft_ms_pu_1v2  "IO8_FT 166MHz HSLV med speed @ 1.2V pullup"
io8_166m_hslv_ft_ms_pd_1v2  "IO8_FT 166MHz HSLV med speed @ 1.2V pulldown"
io8_166m_hslv_ft_ls_1v2  "IO8_FT 166MHz HSLV low speed @ 1.2V"
io8_166m_hslv_ft_ls_pu_1v2  "IO8_FT 166MHz HSLV low speed @ 1.2V pullup"
io8_166m_hslv_ft_ls_pd_1v2  "IO8_FT 166MHz HSLV low speed @ 1.2V pulldown"
io8_166m_hslv_ft_hs_1v8  "IO8_FT 166MHz HSLV high speed @ 1.8V"
io8_166m_hslv_ft_hs_pu_1v8  "IO8_FT 166MHz HSLV high speed @ 1.8V pullup"
io8_166m_hslv_ft_hs_pd_1v8  "IO8_FT 166MHz HSLV high speed @ 1.8V pulldown"
io8_166m_hslv_ft_fs_1v8  "IO8_FT 166MHz HSLV fast speed @ 1.8V"
io8_166m_hslv_ft_fs_pu_1v8  "IO8_FT 166MHz HSLV fast speed @ 1.8V pullup"
io8_166m_hslv_ft_fs_pd_1v8  "IO8_FT 166MHz HSLV fast speed @ 1.8V pulldown"
io8_166m_hslv_ft_ms_1v8  "IO8_FT 166MHz HSLV med speed @ 1.8V"
io8_166m_hslv_ft_ms_pu_1v8  "IO8_FT 166MHz HSLV med speed @ 1.8V pullup"
io8_166m_hslv_ft_ms_pd_1v8  "IO8_FT 166MHz HSLV med speed @ 1.8V pulldown"
io8_166m_hslv_ft_ls_1v8  "IO8_FT 166MHz HSLV low speed @ 1.8V"
io8_166m_hslv_ft_ls_pu_1v8  "IO8_FT 166MHz HSLV low speed @ 1.8V pullup"
io8_166m_hslv_ft_ls_pd_1v8  "IO8_FT 166MHz HSLV low speed @ 1.8V pulldown"
io8_166m_hslv_ft_hs_2v5  "IO8_FT 166MHz HSLV high speed @ 2.5V"
io8_166m_hslv_ft_hs_pu_2v5  "IO8_FT 166MHz HSLV high speed @ 2.5V pullup"
io8_166m_hslv_ft_hs_pd_2v5  "IO8_FT 166MHz HSLV high speed @ 2.5V pulldown"
io8_166m_hslv_ft_fs_2v5  "IO8_FT 166MHz HSLV fast speed @ 2.5V"
io8_166m_hslv_ft_fs_pu_2v5  "IO8_FT 166MHz HSLV fast speed @ 2.5V pullup"
io8_166m_hslv_ft_fs_pd_2v5  "IO8_FT 166MHz HSLV fast speed @ 2.5V pulldown"
io8_166m_hslv_ft_ms_2v5  "IO8_FT 166MHz HSLV med speed @ 2.5V"
io8_166m_hslv_ft_ms_pu_2v5  "IO8_FT 166MHz HSLV med speed @ 2.5V pullup"
io8_166m_hslv_ft_ms_pd_2v5  "IO8_FT 166MHz HSLV med speed @ 2.5V pulldown"
io8_166m_hslv_ft_ls_2v5  "IO8_FT 166MHz HSLV low speed @ 2.5V"
io8_166m_hslv_ft_ls_pu_2v5  "IO8_FT 166MHz HSLV low speed @ 2.5V pullup"
io8_166m_hslv_ft_ls_pd_2v5  "IO8_FT 166MHz HSLV low speed @ 2.5V pulldown"
[Model Selector] io8_166m_hslv_i2c_ft
io8_166m_ft_hs_1v2  "IO8_FT 166MHz high speed @ 1.2V"
io8_166m_ft_hs_pu_1v2  "IO8_FT 166MHz high speed @ 1.2V pullup"
io8_166m_ft_hs_pd_1v2  "IO8_FT 166MHz high speed @ 1.2V pulldown"
io8_166m_ft_fs_1v2  "IO8_FT 166MHz fast speed @ 1.2V"
io8_166m_ft_fs_pu_1v2  "IO8_FT 166MHz fast speed @ 1.2V pullup"
io8_166m_ft_fs_pd_1v2  "IO8_FT 166MHz fast speed @ 1.2V pulldown"
io8_166m_ft_ms_1v2  "IO8_FT 166MHz med speed @ 1.2V"
io8_166m_ft_ms_pu_1v2  "IO8_FT 166MHz med speed @ 1.2V pullup"
io8_166m_ft_ms_pd_1v2  "IO8_FT 166MHz med speed @ 1.2V pulldown"
io8_166m_ft_ls_1v2  "IO8_FT 166MHz low speed @ 1.2V"
io8_166m_ft_ls_pu_1v2  "IO8_FT 166MHz low speed @ 1.2V pullup"
io8_166m_ft_ls_pd_1v2  "IO8_FT 166MHz low speed @ 1.2V pulldown"
io8_166m_ft_hs_1v8  "IO8_FT 166MHz high speed @ 1.8V"
io8_166m_ft_hs_pu_1v8  "IO8_FT 166MHz high speed @ 1.8V pullup"
io8_166m_ft_hs_pd_1v8  "IO8_FT 166MHz high speed @ 1.8V pulldown"
io8_166m_ft_fs_1v8  "IO8_FT 166MHz fast speed @ 1.8V"
io8_166m_ft_fs_pu_1v8  "IO8_FT 166MHz fast speed @ 1.8V pullup"
io8_166m_ft_fs_pd_1v8  "IO8_FT 166MHz fast speed @ 1.8V pulldown"
io8_166m_ft_ms_1v8  "IO8_FT 166MHz med speed @ 1.8V"
io8_166m_ft_ms_pu_1v8  "IO8_FT 166MHz med speed @ 1.8V pullup"
io8_166m_ft_ms_pd_1v8  "IO8_FT 166MHz med speed @ 1.8V pulldown"
io8_166m_ft_ls_1v8  "IO8_FT 166MHz low speed @ 1.8V"
io8_166m_ft_ls_pu_1v8  "IO8_FT 166MHz low speed @ 1.8V pullup"
io8_166m_ft_ls_pd_1v8  "IO8_FT 166MHz low speed @ 1.8V pulldown"
io8_166m_ft_hs_3v3  "IO8_FT 166MHz high speed @ 3.3V"
io8_166m_ft_hs_pu_3v3  "IO8_FT 166MHz high speed @ 3.3V pullup"
io8_166m_ft_hs_pd_3v3  "IO8_FT 166MHz high speed @ 3.3V pulldown"
io8_166m_ft_fs_3v3  "IO8_FT 166MHz fast speed @ 3.3V"
io8_166m_ft_fs_pu_3v3  "IO8_FT 166MHz fast speed @ 3.3V pullup"
io8_166m_ft_fs_pd_3v3  "IO8_FT 166MHz fast speed @ 3.3V pulldown"
io8_166m_ft_ms_3v3  "IO8_FT 166MHz med speed @ 3.3V"
io8_166m_ft_ms_pu_3v3  "IO8_FT 166MHz med speed @ 3.3V pullup"
io8_166m_ft_ms_pd_3v3  "IO8_FT 166MHz med speed @ 3.3V pulldown"
io8_166m_ft_ls_3v3  "IO8_FT 166MHz low speed @ 3.3V"
io8_166m_ft_ls_pu_3v3  "IO8_FT 166MHz low speed @ 3.3V pullup"
io8_166m_ft_ls_pd_3v3  "IO8_FT 166MHz low speed @ 3.3V pulldown"
io8_166m_hslv_ft_hs_1v2  "IO8_FT 166MHz HSLV high speed @ 1.2V"
io8_166m_hslv_ft_hs_pu_1v2  "IO8_FT 166MHz HSLV high speed @ 1.2V pullup"
io8_166m_hslv_ft_hs_pd_1v2  "IO8_FT 166MHz HSLV high speed @ 1.2V pulldown"
io8_166m_hslv_ft_fs_1v2  "IO8_FT 166MHz HSLV fast speed @ 1.2V"
io8_166m_hslv_ft_fs_pu_1v2  "IO8_FT 166MHz HSLV fast speed @ 1.2V pullup"
io8_166m_hslv_ft_fs_pd_1v2  "IO8_FT 166MHz HSLV fast speed @ 1.2V pulldown"
io8_166m_hslv_ft_ms_1v2  "IO8_FT 166MHz HSLV med speed @ 1.2V"
io8_166m_hslv_ft_ms_pu_1v2  "IO8_FT 166MHz HSLV med speed @ 1.2V pullup"
io8_166m_hslv_ft_ms_pd_1v2  "IO8_FT 166MHz HSLV med speed @ 1.2V pulldown"
io8_166m_hslv_ft_ls_1v2  "IO8_FT 166MHz HSLV low speed @ 1.2V"
io8_166m_hslv_ft_ls_pu_1v2  "IO8_FT 166MHz HSLV low speed @ 1.2V pullup"
io8_166m_hslv_ft_ls_pd_1v2  "IO8_FT 166MHz HSLV low speed @ 1.2V pulldown"
io8_166m_hslv_ft_hs_1v8  "IO8_FT 166MHz HSLV high speed @ 1.8V"
io8_166m_hslv_ft_hs_pu_1v8  "IO8_FT 166MHz HSLV high speed @ 1.8V pullup"
io8_166m_hslv_ft_hs_pd_1v8  "IO8_FT 166MHz HSLV high speed @ 1.8V pulldown"
io8_166m_hslv_ft_fs_1v8  "IO8_FT 166MHz HSLV fast speed @ 1.8V"
io8_166m_hslv_ft_fs_pu_1v8  "IO8_FT 166MHz HSLV fast speed @ 1.8V pullup"
io8_166m_hslv_ft_fs_pd_1v8  "IO8_FT 166MHz HSLV fast speed @ 1.8V pulldown"
io8_166m_hslv_ft_ms_1v8  "IO8_FT 166MHz HSLV med speed @ 1.8V"
io8_166m_hslv_ft_ms_pu_1v8  "IO8_FT 166MHz HSLV med speed @ 1.8V pullup"
io8_166m_hslv_ft_ms_pd_1v8  "IO8_FT 166MHz HSLV med speed @ 1.8V pulldown"
io8_166m_hslv_ft_ls_1v8  "IO8_FT 166MHz HSLV low speed @ 1.8V"
io8_166m_hslv_ft_ls_pu_1v8  "IO8_FT 166MHz HSLV low speed @ 1.8V pullup"
io8_166m_hslv_ft_ls_pd_1v8  "IO8_FT 166MHz HSLV low speed @ 1.8V pulldown"
io8_166m_hslv_ft_hs_2v5  "IO8_FT 166MHz HSLV high speed @ 2.5V"
io8_166m_hslv_ft_hs_pu_2v5  "IO8_FT 166MHz HSLV high speed @ 2.5V pullup"
io8_166m_hslv_ft_hs_pd_2v5  "IO8_FT 166MHz HSLV high speed @ 2.5V pulldown"
io8_166m_hslv_ft_fs_2v5  "IO8_FT 166MHz HSLV fast speed @ 2.5V"
io8_166m_hslv_ft_fs_pu_2v5  "IO8_FT 166MHz HSLV fast speed @ 2.5V pullup"
io8_166m_hslv_ft_fs_pd_2v5  "IO8_FT 166MHz HSLV fast speed @ 2.5V pulldown"
io8_166m_hslv_ft_ms_2v5  "IO8_FT 166MHz HSLV med speed @ 2.5V"
io8_166m_hslv_ft_ms_pu_2v5  "IO8_FT 166MHz HSLV med speed @ 2.5V pullup"
io8_166m_hslv_ft_ms_pd_2v5  "IO8_FT 166MHz HSLV med speed @ 2.5V pulldown"
io8_166m_hslv_ft_ls_2v5  "IO8_FT 166MHz HSLV low speed @ 2.5V"
io8_166m_hslv_ft_ls_pu_2v5  "IO8_FT 166MHz HSLV low speed @ 2.5V pullup"
io8_166m_hslv_ft_ls_pd_2v5  "IO8_FT 166MHz HSLV low speed @ 2.5V pulldown"
io8_166m_i2c_ft_1v2  "IO8_FT 166MHz I2C @ 1.2V"
io8_166m_i2c_ft_pu_1v2  "IO8_FT 166MHz I2C @ 1.2V pullup"
io8_166m_i2c_ft_pd_1v2  "IO8_FT 166MHz I2C @ 1.2V pulldown"
io8_166m_i2c_ft_1v8  "IO8_FT 166MHz I2C @ 1.8V"
io8_166m_i2c_ft_pu_1v8  "IO8_FT 166MHz I2C @ 1.8V pullup"
io8_166m_i2c_ft_pd_1v8  "IO8_FT 166MHz I2C @ 1,8V pulldown"
io8_166m_i2c_ft_3v3  "IO8_FT 166MHz I2C @ 3.3V"
io8_166m_i2c_ft_pu_3v3  "IO8_FT 166MHz I2C HSLV @ 3.3V pullup"
io8_166m_i2c_ft_pd_3v3  "IO8_FT 166MHz I2C @ 3.3V pulldown"
[Model Selector] io8_100m_ft_v33
io8_ft_v33_hs_1v2  "IO8_FT_V33 high speed @ 1.2V"
io8_ft_v33_hs_pu_1v2  "IO8_FT_V33 high speed @ 1.2V pullup"
io8_ft_v33_hs_pd_1v2  "IO8_FT_V33 high speed @ 1.2V pulldown"
io8_ft_v33_fs_1v2  "IO8_FT_V33 fast speed @ 1.2V"
io8_ft_v33_fs_pu_1v2  "IO8_FT_V33 fast speed @ 1.2V pullup"
io8_ft_v33_fs_pd_1v2  "IO8_FT_V33 fast speed @ 1.2V pulldown"
io8_ft_v33_ms_1v2  "IO8_FT_V33 med speed @ 1.2V"
io8_ft_v33_ms_pu_1v2  "IO8_FT_V33 med speed @ 1.2V pullup"
io8_ft_v33_ms_pd_1v2  "IO8_FT_V33 med speed @ 1.2V pulldown"
io8_ft_v33_ls_1v2  "IO8_FT_V33 low speed @ 1.2V"
io8_ft_v33_ls_pu_1v2  "IO8_FT_V33 low speed @ 1.2V pullup"
io8_ft_v33_ls_pd_1v2  "IO8_FT_V33 low speed @ 1.2V pulldown"
io8_ft_v33_hs_1v8  "IO8_FT_V33 high speed @ 1.8V"
io8_ft_v33_hs_pu_1v8  "IO8_FT_V33 high speed @ 1.8V pullup"
io8_ft_v33_hs_pd_1v8  "IO8_FT_V33 high speed @ 1.8V pulldown"
io8_ft_v33_fs_1v8  "IO8_FT_V33 fast speed @ 1.8V"
io8_ft_v33_fs_pu_1v8  "IO8_FT_V33 fast speed @ 1.8V pullup"
io8_ft_v33_fs_pd_1v8  "IO8_FT_V33 fast speed @ 1.8V pulldown"
io8_ft_v33_ms_1v8  "IO8_FT_V33 med speed @ 1.8V"
io8_ft_v33_ms_pu_1v8  "IO8_FT_V33 med speed @ 1.8V pullup"
io8_ft_v33_ms_pd_1v8  "IO8_FT_V33 med speed @ 1.8V pulldown"
io8_ft_v33_ls_1v8  "IO8_FT_V33 low speed @ 1.8V"
io8_ft_v33_ls_pu_1v8  "IO8_FT_V33 low speed @ 1.8V pullup"
io8_ft_v33_ls_pd_1v8  "IO8_FT_V33 low speed @ 1.8V pulldown"
io8_ft_v33_hs_3v3  "IO8_FT_V33 high speed @ 3.3V"
io8_ft_v33_hs_pu_3v3  "IO8_FT_V33 high speed @ 3.3V pullup"
io8_ft_v33_hs_pd_3v3  "IO8_FT_V33 high speed @ 3.3V pulldown"
io8_ft_v33_fs_3v3  "IO8_FT_V33 fast speed @ 3.3V"
io8_ft_v33_fs_pu_3v3  "IO8_FT_V33 fast speed @ 3.3V pullup"
io8_ft_v33_fs_pd_3v3  "IO8_FT_V33 fast speed @ 3.3V pulldown"
io8_ft_v33_ms_3v3  "IO8_FT_V33 med speed @ 3.3V"
io8_ft_v33_ms_pu_3v3  "IO8_FT_V33 med speed @ 3.3V pullup"
io8_ft_v33_ms_pd_3v3  "IO8_FT_V33 med speed @ 3.3V pulldown"
io8_ft_v33_ls_3v3  "IO8_FT_V33 low speed @ 3.3V"
io8_ft_v33_ls_pu_3v3  "IO8_FT_V33 low speed @ 3.3V pullup"
io8_ft_v33_ls_pd_3v3  "IO8_FT_V33 low speed @ 3.3V pulldown"
[Define Package Model]  455-wlcsp-56-100mhz-230421
[Manufacturer]  Unknown
[OEM]  Unknown
[Description]  None
[Number Of Pins]  56
[Pin Numbers]
| Pin Num   Terminal Name
E9 | NRST
F10 | PA0
G13 | PA1
E7 | PA2
D6 | PA3
G11 | PA4
F8 | PA5
G9 | PA6
H10 | PA7
E5 | PA8
D2 | PA9
D4 | PA10
C1 | PA11
C3 | PA12
C5 | PA13
A5 | PA14
A3 | PA15
F6 | PB0
F4 | PB1
G7 | PB2
B4 | PB3
B6 | PB4
A7 | PB5
C7 | PB6
D8 | PB7
A9 | PB8
C9 | PB9
E3 | PB12
G1 | PB13
E1 | PB14
F2 | PB15
D12 | PC13
C13 | PC14-OSC32_IN
D14 | PC15-OSC32_OUT
C11 | PE3
B12 | PE4
D10 | PE5
E13 | PH0-OSC_IN
E11 | PH1-OSC_OUT
B8 | PH3-BOOT0
H4 | VDD11
A11 | VDD11
B14 | VBAT
A1 | VDDUSB
A13 | VDD
H2 | VDD
H12 | VDD
F12 | VDDA
H6 | VDDSMPS
H8 | VLXSMPS
B2 | VSS
B10 | VSS
G3 | VSS
H14 | VSS
F14 | VSSA
G5 | VSSSMPS
[Model Data]
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[End Model Data]
[End Package Model]
| Models and submodels in the file (208): io8_100m_ft_hs_1v2 (I/O), io8_100m_ft_hs_pu_1v2 (I/O), io8_100m_ft_hs_pd_1v2 (I/O), io8_100m_ft_fs_1v2 (I/O), io8_100m_ft_fs_pu_1v2 (I/O), io8_100m_ft_fs_pd_1v2 (I/O), io8_100m_ft_ms_1v2 (I/O), io8_100m_ft_ms_pu_1v2 (I/O), io8_100m_ft_ms_pd_1v2 (I/O), io8_100m_ft_ls_1v2 (I/O), io8_100m_ft_ls_pu_1v2 (I/O), io8_100m_ft_ls_pd_1v2 (I/O), io8_100m_ft_hs_1v8 (I/O), io8_100m_ft_hs_pu_1v8 (I/O), io8_100m_ft_hs_pd_1v8 (I/O), io8_100m_ft_fs_1v8 (I/O), io8_100m_ft_fs_pu_1v8 (I/O), io8_100m_ft_fs_pd_1v8 (I/O), io8_100m_ft_ms_1v8 (I/O), io8_100m_ft_ms_pu_1v8 (I/O), io8_100m_ft_ms_pd_1v8 (I/O), io8_100m_ft_ls_1v8 (I/O), io8_100m_ft_ls_pu_1v8 (I/O), io8_100m_ft_ls_pd_1v8 (I/O), io8_100m_ft_hs_3v3 (I/O), io8_100m_ft_hs_pu_3v3 (I/O), io8_100m_ft_hs_pd_3v3 (I/O), io8_100m_ft_fs_3v3 (I/O), io8_100m_ft_fs_pu_3v3 (I/O), io8_100m_ft_fs_pd_3v3 (I/O), io8_100m_ft_ms_3v3 (I/O), io8_100m_ft_ms_pu_3v3 (I/O), io8_100m_ft_ms_pd_3v3 (I/O), io8_100m_ft_ls_3v3 (I/O), io8_100m_ft_ls_pu_3v3 (I/O), io8_100m_ft_ls_pd_3v3 (I/O), io8_100m_hslv_ft_hs_1v2 (I/O), io8_100m_hslv_ft_hs_pu_1v2 (I/O), io8_100m_hslv_ft_hs_pd_1v2 (I/O), io8_100m_hslv_ft_fs_1v2 (I/O), io8_100m_hslv_ft_fs_pu_1v2 (I/O), io8_100m_hslv_ft_fs_pd_1v2 (I/O), io8_100m_hslv_ft_ms_1v2 (I/O), io8_100m_hslv_ft_ms_pu_1v2 (I/O), io8_100m_hslv_ft_ms_pd_1v2 (I/O), io8_100m_hslv_ft_ls_1v2 (I/O), io8_100m_hslv_ft_ls_pu_1v2 (I/O), io8_100m_hslv_ft_ls_pd_1v2 (I/O), io8_100m_hslv_ft_hs_1v8 (I/O), io8_100m_hslv_ft_hs_pu_1v8 (I/O), io8_100m_hslv_ft_hs_pd_1v8 (I/O), io8_100m_hslv_ft_fs_1v8 (I/O), io8_100m_hslv_ft_fs_pu_1v8 (I/O), io8_100m_hslv_ft_fs_pd_1v8 (I/O), io8_100m_hslv_ft_ms_1v8 (I/O), io8_100m_hslv_ft_ms_pu_1v8 (I/O), io8_100m_hslv_ft_ms_pd_1v8 (I/O), io8_100m_hslv_ft_ls_1v8 (I/O), io8_100m_hslv_ft_ls_pu_1v8 (I/O), io8_100m_hslv_ft_ls_pd_1v8 (I/O), io8_100m_hslv_ft_hs_2v5 (I/O), io8_100m_hslv_ft_hs_pu_2v5 (I/O), io8_100m_hslv_ft_hs_pd_2v5 (I/O), io8_100m_hslv_ft_fs_2v5 (I/O), io8_100m_hslv_ft_fs_pu_2v5 (I/O), io8_100m_hslv_ft_fs_pd_2v5 (I/O), io8_100m_hslv_ft_ms_2v5 (I/O), io8_100m_hslv_ft_ms_pu_2v5 (I/O), io8_100m_hslv_ft_ms_pd_2v5 (I/O), io8_100m_hslv_ft_ls_2v5 (I/O), io8_100m_hslv_ft_ls_pu_2v5 (I/O), io8_100m_hslv_ft_ls_pd_2v5 (I/O), io8_166m_ft_hs_1v2 (I/O), io8_166m_ft_hs_pu_1v2 (I/O), io8_166m_ft_hs_pd_1v2 (I/O), io8_166m_ft_fs_1v2 (I/O), io8_166m_ft_fs_pu_1v2 (I/O), io8_166m_ft_fs_pd_1v2 (I/O), io8_166m_ft_ms_1v2 (I/O), io8_166m_ft_ms_pu_1v2 (I/O)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
